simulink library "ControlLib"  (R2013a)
settings: Solver=ode45  StartTime=0.0  StopTime=10.0  RelTol=1e-3
undefined symbols (not defined in the file or in its folder): SimParam

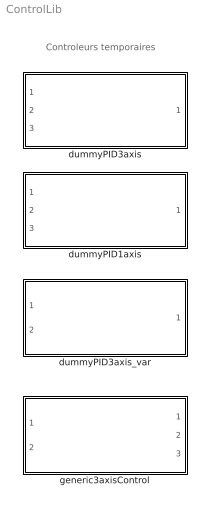
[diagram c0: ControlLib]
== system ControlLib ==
  note: Controleurs temporaires
  dummyPID1axis : Subsystem  InitFcn=SimParam.Control = Control_ParamInitFnc(RawParam,1);  VariantControl=controlVarDefault
  dummyPID3axis : Subsystem  InitFcn=SimParam.Control = Control_ParamInitFnc(RawParam,1);  VariantControl=controlVarDefault
  dummyPID3axis_var : Subsystem  InitFcn=SimParam.Control = Control_ParamInitFnc(RawParam,2);  VariantControl=controlVarDefault
  generic3axisControl : Subsystem  InitFcn=SimParam.Control = GenericControl_ParamInitFnc(RawParam,1);  VariantControl=controlVarDefault

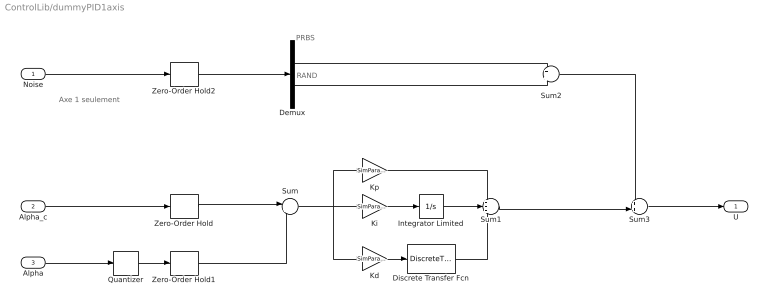
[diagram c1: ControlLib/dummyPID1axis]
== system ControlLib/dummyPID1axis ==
  note: Axe 1 seulement
  note: RAND
  note: PRBS
  Noise : Inport
  Alpha_c : Inport  Port=2
  Alpha : Inport  Port=3
  Demux : Demux  Outputs=2
  Discrete Transfer Fcn : DiscreteTransferFcn  Numerator=[1 0 -1]  Denominator=[2 0 0]
  Integrator Limited : Integrator  LimitOutput=on  UpperSaturationLimit=1  LowerSaturationLimit=-1
  Kd : Gain  Gain=SimParam.Control.Kd/SimParam.Control.Te
  Ki : Gain  Gain=SimParam.Control.Ki*SimParam.Control.Te
  Kp : Gain  Gain=SimParam.Control.Kp
  Quantizer : Quantizer  QuantizationInterval=SimParam.Control.CoderResol
  Sum : Sum  Inputs=|+-
  Sum1 : Sum  Inputs=+++
  Sum2 : Sum  Inputs=+|+
  Sum3 : Sum  Inputs=++|
  Zero-Order Hold : ZeroOrderHold  SampleTime=SimParam.Control.Te
  Zero-Order Hold1 : ZeroOrderHold  SampleTime=SimParam.Control.Te
  Zero-Order Hold2 : ZeroOrderHold  SampleTime=SimParam.Control.Te
  U : Outport
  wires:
  Kd/1 -> Discrete Transfer Fcn/1
  Zero-Order Hold/1 -> Sum/1
  Quantizer/1 -> Zero-Order Hold1/1
  Noise/1 -> Zero-Order Hold2/1
  Discrete Transfer Fcn/1 -> Sum1/3
  Kp/1 -> Sum1/1
  Demux/1 -> Sum2/1
  Ki/1 -> Integrator Limited/1
  Integrator Limited/1 -> Sum1/2
  Sum/1 -> Ki/1, Kp/1, Kd/1
  Zero-Order Hold1/1 -> Sum/2
  Demux/2 -> Sum2/2
  Zero-Order Hold2/1 -> Demux/1
  Alpha_c/1 -> Zero-Order Hold/1
  Alpha/1 -> Quantizer/1
  Sum3/1 -> U/1
  Sum1/1 -> Sum3/2
  Sum2/1 -> Sum3/1

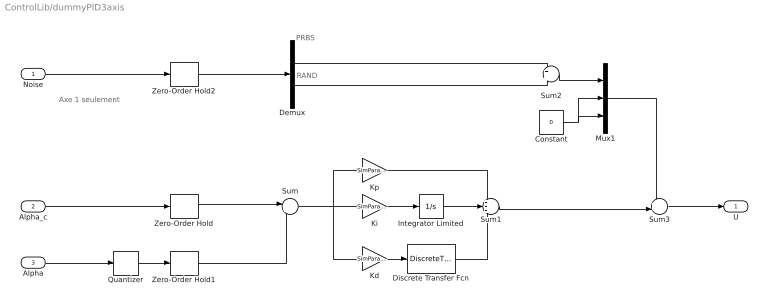
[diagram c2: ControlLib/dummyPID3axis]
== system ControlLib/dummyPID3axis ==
  note: Axe 1 seulement
  note: RAND
  note: PRBS
  Noise : Inport
  Alpha_c : Inport  Port=2
  Alpha : Inport  Port=3
  Constant : Constant  Value=0
  Demux : Demux  Outputs=2
  Discrete Transfer Fcn : DiscreteTransferFcn  Numerator=[1 0 -1]  Denominator=[2 0 0]
  Integrator Limited : Integrator  LimitOutput=on  UpperSaturationLimit=1  LowerSaturationLimit=-1
  Kd : Gain  Gain=SimParam.Control.Kd/SimParam.Control.Te
  Ki : Gain  Gain=SimParam.Control.Ki*SimParam.Control.Te
  Kp : Gain  Gain=SimParam.Control.Kp
  Mux1 : Mux  Inputs=3
  Quantizer : Quantizer  QuantizationInterval=SimParam.Control.CoderResol
  Sum : Sum  Inputs=|+-
  Sum1 : Sum  Inputs=+++
  Sum2 : Sum  Inputs=+|+
  Sum3 : Sum  Inputs=++|
  Zero-Order Hold : ZeroOrderHold  SampleTime=SimParam.Control.Te
  Zero-Order Hold1 : ZeroOrderHold  SampleTime=SimParam.Control.Te
  Zero-Order Hold2 : ZeroOrderHold  SampleTime=SimParam.Control.Te
  U : Outport
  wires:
  Kd/1 -> Discrete Transfer Fcn/1
  Zero-Order Hold/1 -> Sum/1
  Quantizer/1 -> Zero-Order Hold1/1
  Noise/1 -> Zero-Order Hold2/1
  Discrete Transfer Fcn/1 -> Sum1/3
  Kp/1 -> Sum1/1
  Demux/1 -> Sum2/1
  Ki/1 -> Integrator Limited/1
  Integrator Limited/1 -> Sum1/2
  Sum/1 -> Ki/1, Kp/1, Kd/1
  Zero-Order Hold1/1 -> Sum/2
  Demux/2 -> Sum2/2
  Zero-Order Hold2/1 -> Demux/1
  Sum2/1 -> Mux1/1
  Alpha_c/1 -> Zero-Order Hold/1
  Alpha/1 -> Quantizer/1
  Constant/1 -> Mux1/2, Mux1/3
  Sum3/1 -> U/1
  Mux1/1 -> Sum3/1
  Sum1/1 -> Sum3/2

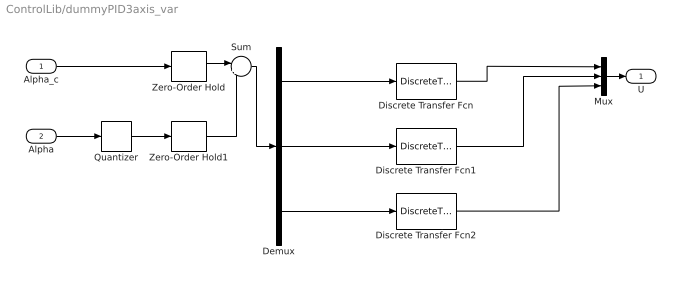
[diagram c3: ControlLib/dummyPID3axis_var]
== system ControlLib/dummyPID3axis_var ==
  Alpha_c : Inport
  Alpha : Inport  Port=2
  Demux : Demux  Outputs=3
  Discrete Transfer Fcn : DiscreteTransferFcn  Numerator=SimParam.Control.KZnum  Denominator=SimParam.Control.KZden
  Discrete Transfer Fcn1 : DiscreteTransferFcn  Numerator=SimParam.Control.KZnum  Denominator=SimParam.Control.KZden
  Discrete Transfer Fcn2 : DiscreteTransferFcn  Numerator=SimParam.Control.KZnum  Denominator=SimParam.Control.KZden
  Mux : Mux  Inputs=3
  Quantizer : Quantizer  QuantizationInterval=SimParam.Control.CoderResol
  Sum : Sum  Inputs=|+-
  Zero-Order Hold : ZeroOrderHold  SampleTime=SimParam.Control.Te
  Zero-Order Hold1 : ZeroOrderHold  SampleTime=SimParam.Control.Te
  U : Outport
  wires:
  Alpha_c/1 -> Zero-Order Hold/1
  Zero-Order Hold1/1 -> Sum/2
  Zero-Order Hold/1 -> Sum/1
  Alpha/1 -> Quantizer/1
  Quantizer/1 -> Zero-Order Hold1/1
  Discrete Transfer Fcn1/1 -> Mux/2
  Demux/2 -> Discrete Transfer Fcn1/1
  Sum/1 -> Demux/1
  Demux/1 -> Discrete Transfer Fcn/1
  Demux/3 -> Discrete Transfer Fcn2/1
  Mux/1 -> U/1
  Discrete Transfer Fcn/1 -> Mux/1
  Discrete Transfer Fcn2/1 -> Mux/3

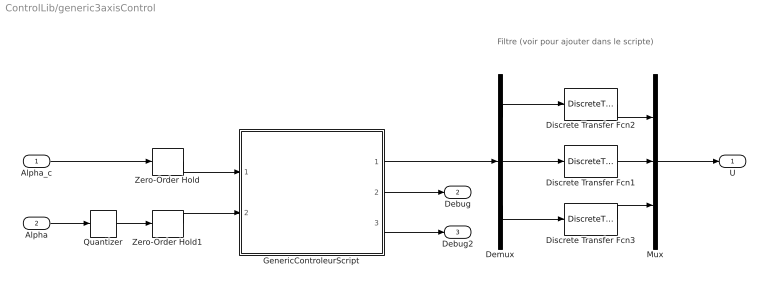
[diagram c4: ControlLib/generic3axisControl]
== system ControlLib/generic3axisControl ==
  note: Filtre (voir pour ajouter dans le scripte)
  Alpha_c : Inport
  Alpha : Inport  Port=2
  Demux : Demux  Outputs=3
  Discrete Transfer Fcn1 : DiscreteTransferFcn  Numerator=SimParam.Control.FZnum  Denominator=SimParam.Control.FZden
  Discrete Transfer Fcn2 : DiscreteTransferFcn  Numerator=SimParam.Control.FZnum  Denominator=SimParam.Control.FZden
  Discrete Transfer Fcn3 : DiscreteTransferFcn  Numerator=SimParam.Control.FZnum  Denominator=SimParam.Control.FZden
  GenericControleurScript : MATLAB Function  RequirementInfo="{}  %GIDa_b7313c75_3339_4613_8ec8_95ef9d80aaac"  TreatAsAtomicUnit=on
  Mux : Mux  Inputs=3
  Quantizer : Quantizer  QuantizationInterval=SimParam.Control.CoderResol
  Zero-Order Hold : ZeroOrderHold  SampleTime=SimParam.Control.Te
  Zero-Order Hold1 : ZeroOrderHold  SampleTime=SimParam.Control.Te
  U : Outport
  Debug : Outport  Port=2
  Debug2 : Outport  Port=3
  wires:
  Alpha_c/1 -> Zero-Order Hold/1
  Zero-Order Hold/1 -> GenericControleurScript/1(alphac)
  Alpha/1 -> Quantizer/1
  Quantizer/1 -> Zero-Order Hold1/1
  Zero-Order Hold1/1 -> GenericControleurScript/2(alpha)
  GenericControleurScript/2(debug) -> Debug/1
  GenericControleurScript/1(u) -> Demux/1
  Demux/3 -> Discrete Transfer Fcn3/1
  Demux/2 -> Discrete Transfer Fcn1/1
  Demux/1 -> Discrete Transfer Fcn2/1
  Discrete Transfer Fcn1/1 -> Mux/2
  Discrete Transfer Fcn2/1 -> Mux/1
  Discrete Transfer Fcn3/1 -> Mux/3
  Mux/1 -> U/1
  GenericControleurScript/3(debug2) -> Debug2/1
